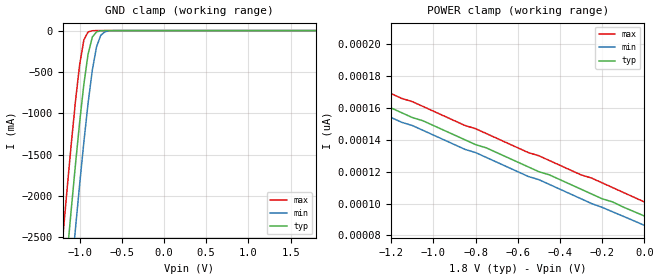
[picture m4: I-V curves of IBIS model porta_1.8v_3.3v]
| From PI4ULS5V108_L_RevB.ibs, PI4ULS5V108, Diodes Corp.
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[Model]   porta_1.8v_3.3v
Model_type Terminator
| variable   typ   min   max
C_comp   3.5236p   3.4973p   3.5489p
[Voltage Range]   1.8000V   1.6200V   1.9800V
[POWER Clamp Reference]   1.8000V   1.6200V   1.9800V
[GND Clamp Reference]   0.0000V   0.0000V   0.0000V
[Temperature Range]   25   85   -40
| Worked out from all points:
|   GND clamp passes 1 mA (typ) near -0.71 V on its own axis
[GND Clamp]
| Voltage   I(typ)   I(min)   I(max)
-1.8V     -10.33A    -11A       -9.655A
-1.2V     -3.313A    -4.105A    -2.505A
-1.15V    -2.735A    -3.53A     -1.931A
-1.1V     -2.17A     -2.959A    -1.377A
-1.05V    -1.624A    -2.401A    -858.9mA
-1V       -1.11A     -1.861A    -410.8mA
-950mV    -647.9mA   -1.348A    -112.9mA
-900mV    -283.7mA   -877.9mA   -15.94mA
-850mV    -78.75mA   -479.3mA   -1.974mA
-800mV    -15.25mA   -197mA     -233.3uA
-700mV    -522.2uA   -13.76mA   -2.027uA
1.8V      92.15pA    96.51pA    91.19pA
[POWER Clamp]
| Voltage   I(typ)   I(min)   I(max)
-1.8V     197pA      173nA      203pA
-1.7V     188pA      6.73nA     197pA
-1.55V    180pA      222pA      189pA
-1.5V     177pA      180pA      186pA
-1.45V    174pA      170pA      183pA
-1.4V     171pA      166pA      181pA
-1.15V    157pA      151pA      166pA
-1.1V     154pA      149pA      164pA
-500mV    120pA      115pA      130pA
-450mV    118pA      112pA      127pA
-250mV    106pA      100pA      116pA
0V        92.2pA     86.3pA     101pA
